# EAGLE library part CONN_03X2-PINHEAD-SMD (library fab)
PIN HEADER
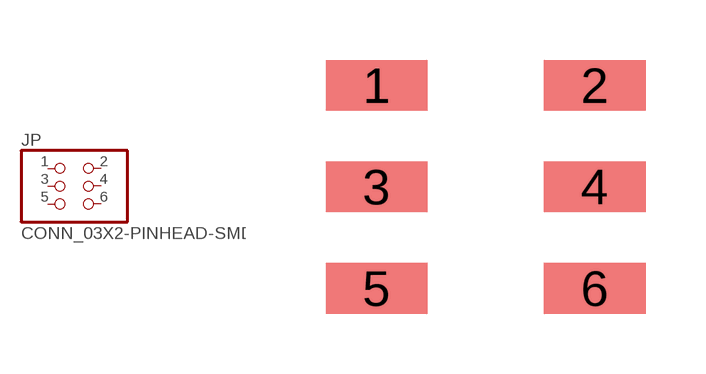
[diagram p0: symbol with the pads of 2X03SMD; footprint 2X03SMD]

Designator prefix JP

## CONN_03X2-PINHEAD-SMD  [2X03SMD]
1  1  pas
2  2  pas
3  3  pas
4  4  pas
5  5  pas
6  6  pas

## Footprint 2X03SMD (pad centres in mm)
smd 2.54 x 1.27: 1 -2.54,2.54; 2 2.92,2.54; 3 -2.54,0; 4 2.92,0; 5 -2.54,-2.54; 6 2.92,-2.54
